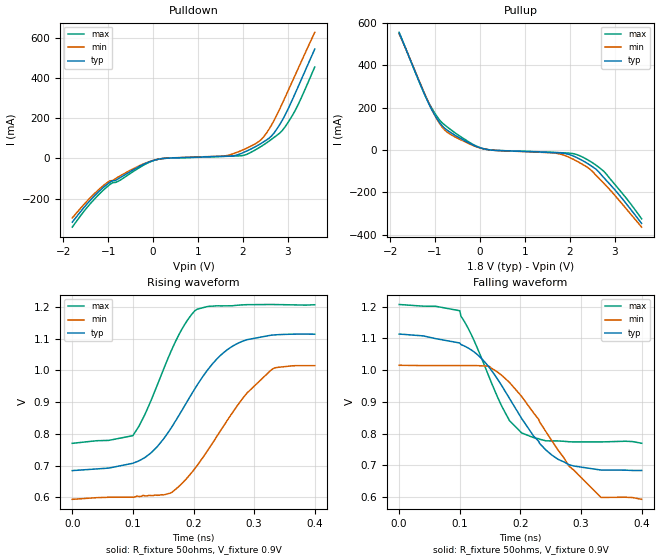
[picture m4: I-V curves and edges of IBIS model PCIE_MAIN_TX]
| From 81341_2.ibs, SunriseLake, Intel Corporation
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[Model]   PCIE_MAIN_TX
Model_type   Output
Polarity   Non-Inverting
|   typ   min   max
C_comp   0.698pF   0.631pF   0.77pF
[Voltage Range]   1.800V   1.620V   1.980V
[Temperature Range]   60.0   110.0   -5.0
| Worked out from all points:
|   slope of the pulldown table from 0 to 0.27 V, typ, clamps not added: 23.8 ohm
|   slope of the pullup table from 0 to 0.27 V, typ, clamps not added: 24.1 ohm
|   rising waveform, R_fixture 50ohms, V_fixture 0.9V: 20-80 % time 90.1ps typ, 92.4ps min, 59ps max; typ from 0.684 V to 1.11 V
|   falling waveform, R_fixture 50ohms, V_fixture 0.9V: 20-80 % time 91.5ps typ, 96.1ps min, 60.4ps max; typ from 1.11 V to 0.684 V
[Pulldown]
|   Voltage   I(typ)   I(min)   I(max)
-1.8V     -316.6mA   -295.3mA   -341.2mA
-1.44V    -217.8mA   -204.6mA   -235.5mA
-1.02V    -127.9mA   -119.7mA   -139.8mA
-60mV     -14.96mA   -13.93mA   -16.33mA
240mV     376.1uA    445.7uA    219.1uA
1.62V     11.2mA     13.45mA    10.65mA
2.04V     32.36mA    46.43mA    16.85mA
2.34V     66.19mA    81.81mA    50.88mA
2.64V     112.3mA    167.1mA    95.75mA
2.94V     216mA      303.8mA    157.4mA
3.24V     361.5mA    451.6mA    272.2mA
3.6V      543.4mA    626.7mA    454.5mA
[Pullup]
|   Voltage   I(typ)   I(min)   I(max)
-1.8V     552.5mA    548.5mA    556.4mA
-1.32V    306.6mA    310.3mA    305.2mA
-1.14V    219mA      222.2mA    223.1mA
-900mV    130.3mA    126mA      141.8mA
-720mV    92.48mA    82.93mA    107.7mA
-180mV    26.1mA     23.7mA     29.48mA
120mV     4.221mA    4.111mA    4.175mA
1.68V     -12.51mA   -14.71mA   -11.32mA
2.16V     -36mA      -52.71mA   -21.63mA
2.46V     -72.27mA   -92.38mA   -53.92mA
2.76V     -131mA     -157.4mA   -100.9mA
3.6V      -346.8mA   -364.4mA   -325.1mA
[Ramp]
| variable   typ   min   max
dV/dt_r   0.307/8.8859e-11 0.300/1.13715e-10 0.311/7.29426e-11
dV/dt_f   0.306/8.98485e-11 0.302/1.15352e-10 0.309/7.35806e-11
R_load = 50ohms
[Rising Waveform]
R_fixture = 50ohms
V_fixture = 0.9V
V_fixture_min = 0.81V
V_fixture_max = 0.99V
|   Time   V(typ)   V(min)   V(max)
0s        684mV      593.4mV    770mV
100ps     707.1mV    600.1mV    794.3mV
130ps     740.1mV    605.1mV    905.4mV
162ps     815.3mV    613.1mV    1.056V
186ps     890.6mV    653.5mV    1.147V
206ps     953.7mV    700.1mV    1.193V
260ps     1.071V     854.9mV    1.204V
288ps     1.097V     928.2mV    1.207V
328ps     1.111V     1.001V     1.208V
400ps     1.114V     1.015V     1.207V
[Falling Waveform]
R_fixture = 50ohms
V_fixture = 0.9V
V_fixture_min = 0.81V
V_fixture_max = 0.99V
|   Time   V(typ)   V(min)   V(max)
0s        1.114V     1.016V     1.207V
100ps     1.086V     1.015V     1.187V
148ps     1.01V      1.013V     980.7mV
182ps     911.3mV    961.6mV    841.3mV
202ps     848.2mV    917.7mV    802.6mV
232ps     768.8mV    836.2mV    782.6mV
262ps     719.6mV    748.9mV    777.4mV
280ps     702.6mV    698.2mV    774.8mV
333ps     685.6mV    599.3mV    774.2mV
400ps     684.3mV    593.4mV    770mV
